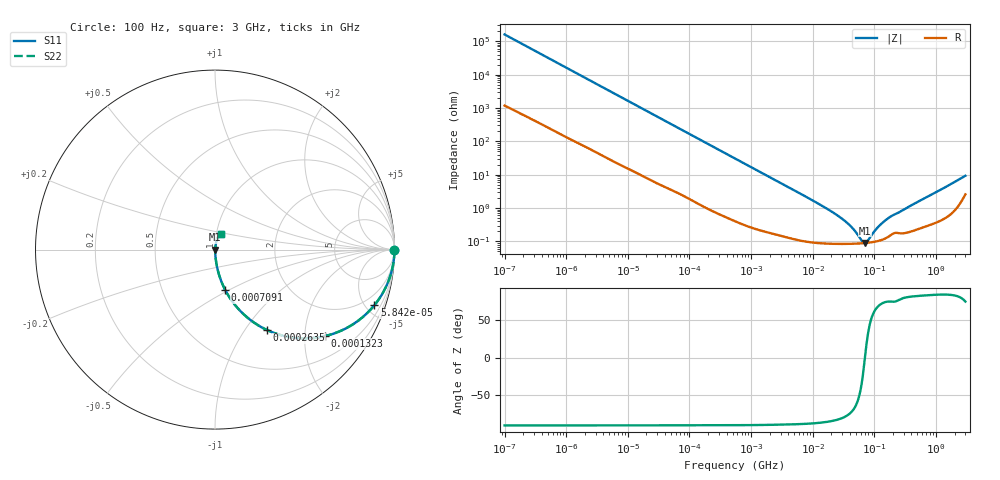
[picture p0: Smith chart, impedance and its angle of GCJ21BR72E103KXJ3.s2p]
!Murata Part Number: GCJ21BR72E103KXJ3
!These Parameters are Measured in Series Mode Connection
!Data Generated on Mar 13, 2026
!  o--ll--o
!Port1  Port2
!  o------o
!Operation Temp=25[degC], DC Bias Voltage=0[V]
!Freq. Start=100[Hz] Stop=3[GHz] 401[Steps]
# Hz S RI R 50
!Freq.(Hz) S11(Real) S11(Imag) S21(Real) S21(Imag) S12(Real) S12(Imag) S22(Real) S22(Imag)
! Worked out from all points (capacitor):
!   401 points, 100 Hz to 3 GHz, reference 50 ohm
!   read as one part in series: C = 9.92 nF near 109 Hz
!   lowest |Z| = 89.7 mohm at 70.93 MHz (marker M1)
!   series resonance near 70.33 MHz, so ESL is about 520 pH
!   S11 on the Smith chart (normalised r, x): 100 Hz: open; 58.42 kHz: 1.06, -5.69; 132.3 kHz: 1.03, -2.53; 263.5 kHz: 1.01, -1.27; 709.1 kHz: 1.01, -0.48; 3 GHz: 1.05, +0.18
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100  1 -0.000624  5e-06 0.000624  5e-06 0.000624  1 -0.000624
1788  0.9998 -0.011  0.000215 0.011  0.000215 0.011  0.9998 -0.011
10003  0.9957 -0.0606  0.00425 0.0606  0.00425 0.0606  0.9957 -0.0606
31977  0.9623 -0.1856  0.0377 0.1856  0.0377 0.1856  0.9623 -0.1856
58416  0.8873 -0.3108  0.1127 0.3108  0.1127 0.3108  0.8873 -0.3108
86054  0.7869 -0.404  0.2131 0.404  0.2131 0.404  0.7869 -0.404
132342  0.6135 -0.4814  0.3865 0.4814  0.3865 0.4814  0.6135 -0.4814
186741  0.4465 -0.4916  0.5535 0.4916  0.5535 0.4916  0.4465 -0.4916
263501  0.2909 -0.4485  0.7091 0.4485  0.7091 0.4485  0.2909 -0.4485
547723  0.0897 -0.2792  0.9103 0.2792  0.9103 0.2792  0.0897 -0.2792
709116  0.0565 -0.2241  0.9435 0.2241  0.9435 0.2241  0.0565 -0.2241
2079876  0.00837 -0.0809  0.9916 0.0809  0.9916 0.0809  0.00837 -0.0809
9794414  0.00123 -0.0172  0.9988 0.0172  0.9988 0.0172  0.00123 -0.0172
1.950129e7  0.000918 -0.00815  0.9991 0.00815  0.9991 0.00815  0.000918 -0.00815
3.131008e7  0.000862 -0.00441  0.9991 0.00441  0.9991 0.00441  0.000862 -0.00441
4.418008e7  0.000857 -0.00236  0.9991 0.00236  0.9991 0.00236  0.000857 -0.00236
6.234031e7  0.000878 -0.000592  0.9991 0.000592  0.9991 0.000592  0.000878 -0.000592
7.093284e7  0.000895 4.27e-05  0.9991 -4.27e-05  0.9991 -4.27e-05  0.000895 4.27e-05
7.730952e7  0.00091 0.000465  0.9991 -0.000465  0.9991 -0.000465  0.00091 0.000465
1.188943e8  0.00105 0.00269  0.9989 -0.00269  0.9989 -0.00269  0.00105 0.00269
1.751444e8  0.00147 0.00505  0.9985 -0.00505  0.9985 -0.00505  0.00147 0.00505
3e9  0.0325 0.0844  0.9675 -0.0844  0.9675 -0.0844  0.0325 0.0844
